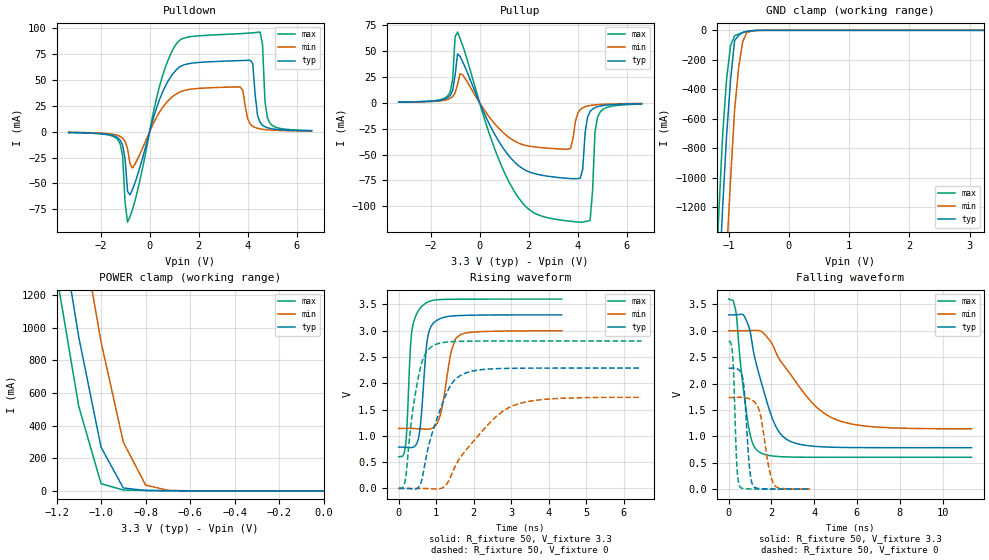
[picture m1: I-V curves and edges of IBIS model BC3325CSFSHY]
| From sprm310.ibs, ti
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|   Model Cell BC3325CSFSHY
|BC3325CSFSHY
[Model]   BC3325CSFSHY
Model_type   I/O
Polarity   Non-Inverting
Enable   Active-Low
Vinl =  0.8v
Vinh =  2v
Cref =  15.0000pF
Rref =  100.0000M
Vref =  0V
Vmeas =  1.65
C_comp   2.5107p   2.136p   3.1702p
[Model Spec]
Vinl   0.8v   0.8v   0.8v
Vinh   2v   2v   2v
[Temperature Range]   25   125   -40
[Voltage Range]   3.3   3   3.6
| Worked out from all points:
|   slope of the pulldown table from 0 to 0.495 V, typ, clamps not added: 13.6 ohm
|   slope of the pullup table from 0 to 0.495 V, typ, clamps not added: 19.6 ohm
|   GND clamp passes 1 mA (typ) near -0.55 V on its own axis
|   POWER clamp passes 1 mA (typ) near -0.67 V on its own axis
|   rising waveform, R_fixture 50, V_fixture 3.3: 20-80 % time 166ps typ, 262ps min, 132ps max; typ from 0.785 V to 3.3 V
|   rising waveform, R_fixture 50, V_fixture 0: 20-80 % time 593ps typ, 1.17ns min, 326ps max; typ from 0 V to 2.29 V
|   falling waveform, R_fixture 50, V_fixture 3.3: 20-80 % time 1.01ns typ, 2.04ns min, 500ps max; typ from 3.3 V to 0.785 V
|   falling waveform, R_fixture 50, V_fixture 0: 20-80 % time 226ps typ, 417ps min, 143ps max; typ from 2.29 V to 0.001 V
[POWER_clamp]
|   voltage   I(typ)   I(min)   I(max)
-3.3V     22.13A     22.81A     21.76A
-1.2V     1.777A     2.558A     1.326A
-1.167V   1.499A     2.271A     1.056A
-1.133V   1.22A      1.985A     786.7mA
-1.1V     941.2mA    1.698A     517.1mA
-1.067V   716.7mA    1.436A     359.5mA
-1.033V   492.1mA    1.174A     201.9mA
-1V       267.6mA    912.1mA    44.33mA
-900mV    17.82mA    298mA      5.452mA
-800mV    2.597mA    36.49mA    3.097mA
-700mV    1.195mA    3.384mA    1.505mA
-11.55fV  42.07pA    6.145nA    501.8fA
[Pulldown]
|   voltage   I(typ)   I(min)   I(max)
-3.3V     -841.7uA   -670.2uA   -911.7uA
-1.3V     -5.852mA   -3.631mA   -7.719mA
-1.1V     -12.99mA   -6.251mA   -23.51mA
-900mV    -57.7mA    -16.72mA   -87.34mA
-700mV    -55.82mA   -35.09mA   -75.1mA
1.1V      59.92mA    36.57mA    85.06mA
3.7V      68.51mA    42.93mA    94.48mA
4.1V      68.8mA     7.362mA    95.13mA
4.5V      8.911mA    2.645mA    95.99mA
4.7V      4.671mA    1.979mA    28.88mA
4.9V      3.124mA    1.577mA    8.243mA
6.6V      798.5uA    571.1uA    1.034mA
[Pullup]
|   voltage   I(typ)   I(min)   I(max)
-3.3V     669.2uA    562.7uA    746.5uA
-1.3V     4.957mA    3.263mA    6.677mA
-1.1V     12mA       5.961mA    22.79mA
-1V       26.99mA    9.54mA     64.01mA
-900mV    47.32mA    18.06mA    68.43mA
1.5V      -59.02mA   -37.99mA   -88.89mA
3.7V      -73.26mA   -44.09mA   -114.6mA
4.1V      -72.88mA   -6.563mA   -115.5mA
4.5V      -8.454mA   -2.591mA   -113.8mA
4.7V      -4.668mA   -1.97mA    -28.57mA
4.9V      -3.189mA   -1.585mA   -9.198mA
6.6V      -843.6uA   -589.3uA   -1.225mA
[GND_clamp]
|   voltage   I(typ)   I(min)   I(max)
-3.3V     -22.45A    -23.24A    -22.02A
-1.233V   -2.371A    -3.249A    -1.858A
-1.167V   -1.783A    -2.654A    -1.277A
-1.1V     -1.21A     -2.069A    -720.1mA
-1.033V   -714.5mA   -1.52A     -330.7mA
-966.7mV  -334.2mA   -1.01A     -102.9mA
-900mV    -69.08mA   -538.8mA   -36.75mA
-833.3mV  -34.64mA   -254mA     -25.31mA
-766.7mV  -14mA      -79.19mA   -15.48mA
-700mV    -7.155mA   -14.42mA   -7.256mA
-433.3mV  -74.68uA   -265.5uA   -24.2uA
3.233V    39.33pA    1.425uA    430.8fA
[Ramp]
| variable   typ   min   max
dV/dt_f   1.515991/1.009533n   1.12013/2.04954n   1.808005/0.5004888n
dV/dt_r   1.381521/0.5938833n   1.048348/1.17704n   1.69071/0.3261254n
R_load = 50
[Rising Waveform]
R_fixture = 50
V_fixture = 3.3
V_fixture_min = 3
V_fixture_max = 3.6
|   time   V(typ)   V(min)   V(max)
0s        785.3mV    1.141V     603.3mV
184ps     782.3mV    1.142V     827.8mV
368ps     780mV      1.14V      3.068V
528ps     954.6mV    1.135V     3.38V
632ps     1.65V      1.13V      3.472V
784ps     2.913V     1.126V     3.546V
1.04ns    3.205V     1.261V     3.588V
1.4ns     3.276V     2.606V     3.596V
1.648ns   3.287V     2.925V     3.597V
4.344ns   3.299V     2.997V     3.6V
[Rising Waveform]
R_fixture = 50
V_fixture = 0
V_fixture_min = 0
V_fixture_max = 0
|   time   V(typ)   V(min)   V(max)
0s        58.73pV    18.5nV     1.577pV
184ps     520.9uV    135.7uV    188.2mV
344ps     -7.479mV   293.3uV    1.315V
552ps     44.2mV     437.1uV    2.207V
912ps     1.096V     -7.846mV   2.711V
1.416ns   1.996V     278.2mV    2.79V
1.888ns   2.217V     809.8mV    2.8V
2.624ns   2.277V     1.383V     2.802V
3.264ns   2.285V     1.623V     2.803V
6.472ns   2.288V     1.732V     2.803V
[Falling Waveform]
R_fixture = 50
V_fixture = 3.3
V_fixture_min = 3
V_fixture_max = 3.6
|   time   V(typ)   V(min)   V(max)
0s        3.3V       3V         3.6V
352ps     3.303V     3V         3.327V
768ps     3.248V     3.002V     1.641V
1.088ns   2.786V     3.005V     906.7mV
1.44ns    2.148V     3.002V     703.1mV
2.184ns   1.204V     2.616V     622.8mV
3.04ns    881.4mV    2.089V     607.2mV
4.208ns   805.6mV    1.517V     603.8mV
5.4ns     790mV      1.266V     603.3mV
11.36ns   785.4mV    1.144V     603.3mV
[Falling Waveform]
R_fixture = 50
V_fixture = 0
V_fixture_min = 0
V_fixture_max = 0
|   time   V(typ)   V(min)   V(max)
0s        2.289V     1.735V     2.803V
184ps     2.292V     1.736V     2.544V
392ps     2.279V     1.739V     387.6mV
536ps     2.237V     1.74V      41mV
712ps     1.942V     1.736V     10.23mV
952ps     500.8mV    1.713V     5.002mV
1.144ns   64.26mV    1.672V     3.464mV
1.472ns   10.18mV    1.43V      2.135mV
2.144ns   2.961mV    74.21mV    824.5uV
3.808ns   743.3uV    3.026mV    141.1uV
